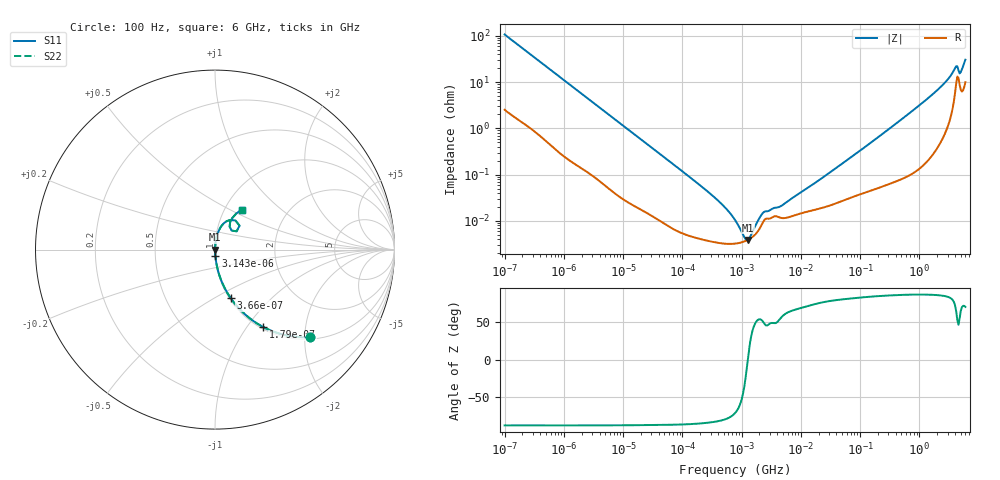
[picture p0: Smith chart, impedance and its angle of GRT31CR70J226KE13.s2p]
!Murata Part Number: GRT31CR70J226KE13
!These Parameters are Measured in Series Mode Connection
!Data Generated on Jun 19, 2026
!  o--ll--o
!Port1  Port2
!  o------o
!Operation Temp=25[degC], DC Bias Voltage=0[V]
!Freq. Start=100[Hz] Stop=6[GHz] 401[Steps]
# Hz S RI R 50
!Freq.(Hz) S11(Real) S11(Imag) S21(Real) S21(Imag) S12(Real) S12(Imag) S22(Real) S22(Imag)
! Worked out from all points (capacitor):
!   401 points, 100 Hz to 6 GHz, reference 50 ohm
!   read as one part in series: C = 14.9 uF near 109 Hz
!   lowest |Z| = 3.88 mohm at 1.268 MHz (marker M1)
!   series resonance near 1.274 MHz, so ESL is about 1.1 nH
!   S11 on the Smith chart (normalised r, x): 100 Hz: 1.05, -2.13; 179 Hz: 1.03, -1.20; 366 Hz: 1.01, -0.59; 3.143 kHz: 1.00, -0.07; 6 GHz: 1.20, +0.57
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100  0.5317 -0.4873  0.4683 0.4873  0.4683 0.4873  0.5317 -0.4873
179  0.2702 -0.432  0.7298 0.432  0.7298 0.432  0.2702 -0.432
366  0.0868 -0.2693  0.9132 0.2693  0.9132 0.2693  0.0868 -0.2693
820  0.0206 -0.1312  0.9794 0.1312  0.9794 0.1312  0.0206 -0.1312
2008  0.00441 -0.0552  0.9956 0.0552  0.9956 0.0552  0.00441 -0.0552
3143  0.00219 -0.0356  0.9978 0.0356  0.9978 0.0356  0.00219 -0.0356
40335  0.000111 -0.0029  0.9999 0.0029  0.9999 0.0029  0.000111 -0.0029
330837  3.53e-05 -0.000342  1 0.000342  1 0.000342  3.53e-05 -0.000342
517687  3.23e-05 -0.000197  1 0.000197  1 0.000197  3.23e-05 -0.000197
774597  3.24e-05 -0.0001  1 0.0001  1 0.0001  3.24e-05 -0.0001
885955  3.32e-05 -7.19e-05  1 7.19e-05  1 7.19e-05  3.32e-05 -7.19e-05
1267578  3.88e-05 -9e-07  1 9e-07  1 9e-07  3.88e-05 -9e-07
1813585  5.61e-05 7.23e-05  0.9999 -7.23e-05  0.9999 -7.23e-05  5.61e-05 7.23e-05
2372521  0.000101 0.000118  0.9999 -0.000118  0.9999 -0.000118  0.000101 0.000118
4643984  0.000116 0.000175  0.9999 -0.000175  0.9999 -0.000175  0.000116 0.000175
1.555665e7  0.000169 0.000577  0.9998 -0.000577  0.9998 -0.000577  0.000169 0.000577
3.124326e8  0.000724 0.00981  0.9993 -0.00981  0.9993 -0.00981  0.000724 0.00981
1.873145e9  0.00698 0.0609  0.993 -0.0609  0.993 -0.0609  0.00698 0.0609
3.205649e9  0.0282 0.1194  0.9718 -0.1194  0.9718 -0.1194  0.0282 0.1194
4.009986e9  0.0844 0.1654  0.9156 -0.1654  0.9156 -0.1654  0.0844 0.1654
5.016141e9  0.0814 0.1282  0.9186 -0.1282  0.9186 -0.1282  0.0814 0.1282
6e9  0.1487 0.2225  0.8513 -0.2225  0.8513 -0.2225  0.1487 0.2225
